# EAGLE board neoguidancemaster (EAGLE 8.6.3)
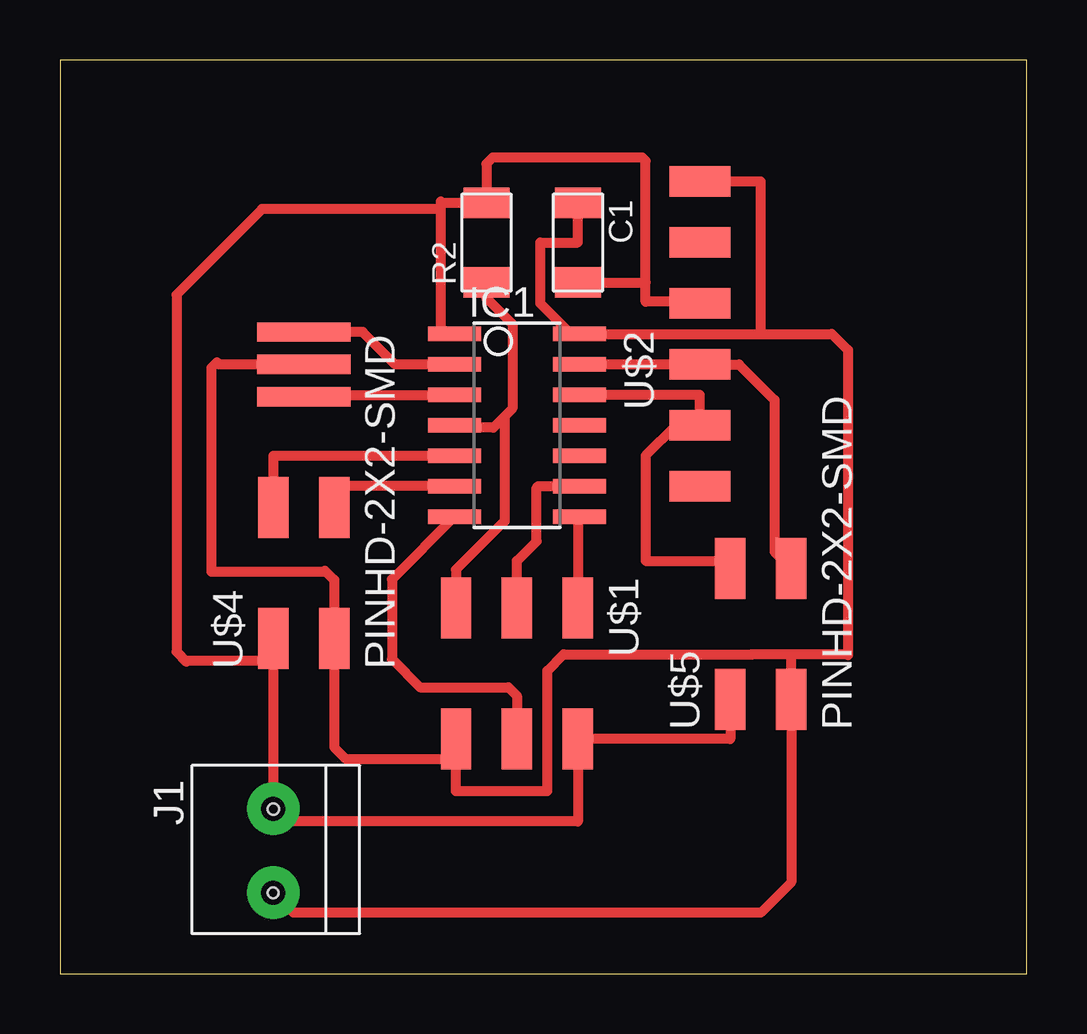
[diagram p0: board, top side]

Size 40.31 x 38.09 mm. Coordinates in mm from the lower left corner, seen from the top.
Outline: 0,0 40.31,0 40.31,38.09 0,38.09 0,0
Copper layers (1*16): Top 0.035mm / dielectric 1.5mm / Bottom 0.035mm
Design rules "rules": minimum track width 16mil, minimum drill 0.8mm, track to track 16mil, track to pad 16mil, pad to pad 16mil, via to via 16mil, smd to smd 16mil, copper to edge 40mil, drill to drill 6mil, minimum pad ring 10mil, minimum via ring 8mil, stop-mask expansion 4mil, vias tented up to drill 0mil, thermal gap 10mil
Holes 0.45 mm at 8.9,6.86 8.89,3.37

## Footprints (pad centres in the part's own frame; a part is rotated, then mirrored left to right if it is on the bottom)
C1206FAB = smd 1.27 x 1.905: 1 -1.651,0; 2 1.651,0
SOIC14 = smd 0.61 x 2.21: 1 -3.81,-2.603; 2 -2.54,-2.603; 3 -1.27,-2.603; 4 0,-2.603; 5 1.27,-2.603; 6 2.54,-2.603; 7 3.81,-2.603; 8 3.81,2.603; 9 2.54,2.603; 10 1.27,2.603; 11 0,2.603; 12 -1.27,2.603; 13 -2.54,2.603; 14 -3.81,2.603
3.5MMTERM = drill 1 pad 2.184: 1 1.8,0; 2 -1.7,0
R1206FAB = smd 1.27 x 1.905: 1 -1.651,0; 2 1.651,0
2X03SMD = smd 2.54 x 1.27: 1 -2.54,2.54; 2 2.92,2.54; 3 -2.54,0; 4 2.92,0; 5 -2.54,-2.54; 6 2.92,-2.54
1X06SMD = smd 2.54 x 1.27: 1 0,6.35; 2 0,3.81; 3 0,1.27; 4 0,-1.27; 5 0,-3.81; 6 0,-6.35
EFOBM = smd 0.8 x 3.9: 1 -1.35,0; 2 0,0; 3 1.35,0
2X02SMD = smd 2.54 x 1.27: 1 -2.54,1.27; 2 2.92,1.27; 3 -2.54,-1.27; 4 2.92,-1.27

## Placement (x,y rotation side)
C1  1UF  [C1206FAB]  21.59,30.48 270 top
IC1  ATTINY44-SSU  [SOIC14]  19.05,22.86 270 top
J1  TERM-1X02-ADAFRUIT  [3.5MMTERM]  8.89,5.08 90 top
R2  10K  [R1206FAB]  17.78,30.48 90 top
U$1  AVRISPSMD  [2X03SMD]  19.05,12.7 270 top
U$2  FTDI-SMD-HEADER  [1X06SMD]  26.67,26.67 0 top
U$3  RESONATOR  [EFOBM]  10.16,25.4 270 top
U$4  PINHD-2X2-SMD  [2X02SMD]  10.16,16.51 90 top
U$5  PINHD-2X2-SMD  [2X02SMD]  29.21,13.97 90 top

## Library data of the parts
C1 IC1 J1 R2 U$1-U$5 = fab

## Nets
A0: IC1.5 U$4.2
GND: C1.1 IC1.14 J1.2 U$1.6 U$2.1 U$3.2 U$4.3 U$5.3
MISO: IC1.8 U$1.1
MOSI: IC1.7 U$1.4
R1: IC1.10
R2: IC1.11
R3: IC1.6 U$4.4
RESET: IC1.4 R2.1 U$1.5
RXD: IC1.12 U$2.5 U$5.2
SCK: IC1.9 U$1.3
TXD: IC1.13 U$2.4 U$5.4
VCC: C1.2 IC1.1 J1.1 R2.2 U$1.2 U$2.3 U$4.1 U$5.1
XTAL1: IC1.2 U$3.1
XTAL2: IC1.3 U$3.3

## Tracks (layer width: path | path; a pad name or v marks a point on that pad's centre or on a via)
A0
  Top 0.406: 17.35,21.59 IC1.5 8.89,21.59 U$4.2
GND
  Top 0.406: 11.43,25.4 U$3.2 6.63,25.4 6.54,25.49 6.31,25.26 6.31,16.76 10.99,16.76 11.04,16.8 11.43,16.41 U$4.3 11.43,9.44 11.91,8.96 16.15,8.96 16.51,9.32 | C1.1 21.59,30.48 20.03,30.48 20.03,27.94 21.3,26.67 IC1.14 29.21,26.67 | 29.21,26.67 29.21,33.02 U$2.1 | 16.51,9.32 16.51,7.62 20.32,7.62 20.32,12.63 21,13.31 28.83,13.31 | 16.51,9.32 U$1.6 | J1.2 9.73,2.54 29.21,2.54 30.48,3.81 U$5.3 30.48,13.22 30.57,13.31 | 28.83,13.31 28.85,13.29 | 29.21,26.67 32.17,26.67 32.85,26 32.85,13.27 32.81,13.31 30.57,13.31 | 30.57,13.31 28.83,13.31
MISO
  Top 0.406: IC1.8 21.59,18.99 U$1.1
MOSI
  Top 0.406: IC1.7 13.83,16.44 13.83,13.12 15.01,11.94 18.69,11.94 19.05,11.58 U$1.4
R3
  Top 0.406: IC1.6 11.4,20.32 11.35,20.27 11.43,20.2 U$4.4
RESET
  Top 0.406: U$1.5 16.51,16.84 18.54,18.87 18.54,23.23 | R2.1 17.78,28.17 18.86,27.09 18.86,23.56 18.54,23.23 | 18.54,23.23 18.07,22.77 16.54,22.77 IC1.4
RXD
  Top 0.406: IC1.12 26.67,24.13 U$2.5 25.68,22.86 24.41,21.59 24.41,17.21 27.62,17.21 U$5.2
SCK
  Top 0.406: U$1.3 19.05,17.21 19.87,18.02 19.87,20.26 19.93,20.32 IC1.9
TXD
  Top 0.406: IC1.13 U$2.4 28.31,25.4 29.79,23.92 29.79,17.58 U$5.4
VCC
  Top 0.152: IC1.1 16.33,26.67 15.87,27.14
  Top 0.406: U$5.1 27.94,9.78 U$1.2 21.59,6.35 9.42,6.35 J1.1 8.89,13.05 | U$4.1 8.89,13.05 | 15.87,31.87 15.87,32.2 15.94,32.13 R2.2 17.78,33.76 18.04,34.02 24.27,34.02 24.41,33.88 24.41,28.82 | 15.87,31.87 15.87,27.14 15.87,26.85 15.68,26.66 | 15.87,31.87 8.42,31.87 4.85,28.31 4.85,13.42 5.28,13 5.32,13.05 8.89,13.05 | U$2.3 26.6,28.01 24.41,28.01 24.41,28.82 | C1.2 21.6,28.82 24.41,28.82
XTAL1
  Top 0.406: IC1.2 13.97,25.4 12.62,26.75 U$3.1
XTAL2
  Top 0.406: U$3.3 10.24,24.13 IC1.3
